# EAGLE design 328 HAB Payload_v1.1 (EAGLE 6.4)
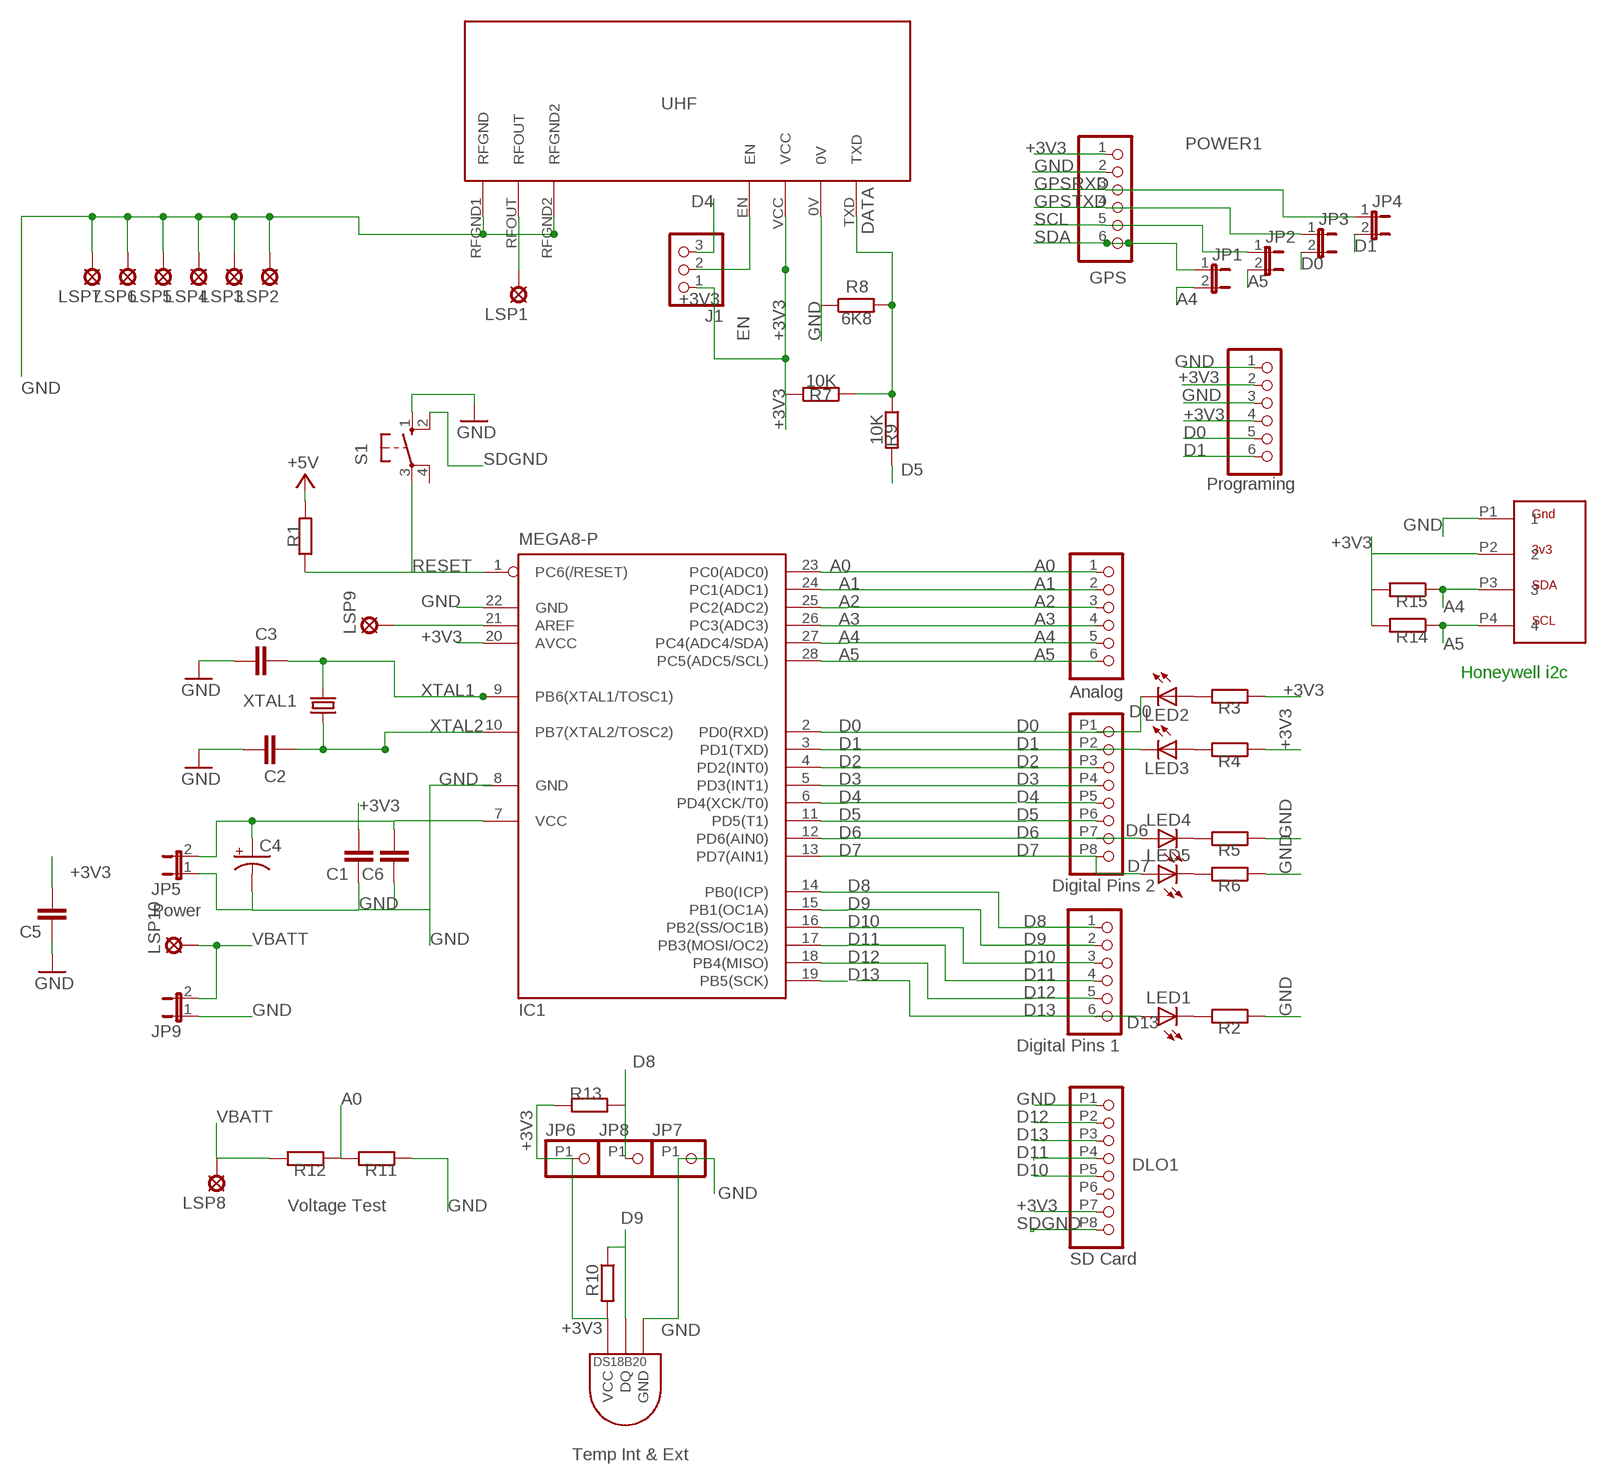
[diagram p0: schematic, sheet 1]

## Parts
ANALOG  PINHD-1X6CLEAN  [1X06-CLEAN]
C1  C-EU025-025X050  [C025-025X050]
C2  C-EU025-025X050  [C025-025X050]
C3  C-EU025-025X050  [C025-025X050]
C4  CAP_POLPTH4  [CPOL-RADIAL-1000UF-25V]
C5  C-EU025-025X050  [C025-025X050]
C6  C-EU025-025X050  [C025-025X050]
DHI  PINHD-1X6CLEAN  [1X06-CLEAN]
DLO  PINHD-1X8  [1X08SMALL]
DLO1  PINHD-1X8  [1X08SMALL]
IC1  MEGA8-P  [DIL28-3]
J1  PINHD-1X3CB  [1X03-CLEANBIG]
JP1  JUMPER-2PTH  [1X02]
JP2  JUMPER-2PTH  [1X02]
JP3  JUMPER-2PTH  [1X02]
JP4  JUMPER-2PTH  [1X02]
JP5  JUMPER-2PTH  [1X02]
JP6  PINHD-1X1UGI  [1X01SML-SQR]
JP7  PINHD-1X1UGI  [1X01SML-SQR]
JP8  PINHD-1X1UGI  [1X01SML-SQR]
JP9  JUMPER-2PTH  [1X02]
LED1  LED3MM  [LED3MM]
LED2  LED3MM  [LED3MM]
LED3  LED3MM  [LED3MM]
LED4  LED3MM  [LED3MM]
LED5  LED3MM  [LED3MM]
LSP1  LSP10  [LSP10]
LSP2  LSP10  [LSP10]
LSP3  LSP13  [LSP13]
LSP4  LSP13  [LSP13]
LSP5  LSP13  [LSP13]
LSP6  LSP13  [LSP13]
LSP7  LSP10  [LSP10]
LSP8  LSP10  [LSP10]
LSP9  LSP10  [LSP10]
LSP10  LSP10  [LSP10]
POWER  PINHD-1X6CLEAN  [1X06-CLEAN]
POWER1  PINHD-1X6CLEAN  [1X06-CLEAN]
R1  R-EU_0207/2V  [0207/2V]
R2  R-EU_0207/2V  [0207/2V]
R3  R-EU_0207/2V  [0207/2V]
R4  R-EU_0207/2V  [0207/2V]
R5  R-EU_0207/2V  [0207/2V]
R6  R-EU_0207/2V  [0207/2V]
R7  10K  R-EU_0207/2V  [0207/2V]
R8  6K8  R-EU_0207/2V  [0207/2V]
R9  10K  R-EU_0207/2V  [0207/2V]
R10  R-EU_0207/2V  [0207/2V]
R11  R-EU_0207/2V  [0207/2V]
R12  R-EU_0207/2V  [0207/2V]
R13  R-EU_0207/2V  [0207/2V]
R14  R-EU_0207/2V  [0207/2V]
R15  R-EU_0207/2V  [0207/2V]
S1  10-XX  [B3F-10XX]
U$1  NTX2-VERTICAL  [NTX2-VERTICAL]
U$2  HSCDANN001BA2A3  [HDC-DIL8]
U$3  DS1820TO92  [DS1820]
XTAL1  CRYTALHC49S  [HC49/S]

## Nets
+3V3 [usbvcc]: C1.2 C4.1(+) C5.2 C6.2 DLO1.P7 IC1.7(VCC) IC1.20(AVCC) J1.1 JP5.2 JP6.P1 POWER1.1 POWER.2 POWER.4 R1.2 R3.1 R4.1 R7.2 R10.2 R13.1 R14.2 R15.2 U$1.VCC U$2.P2 U$3.VDD(VCC) ; supply symbol labelled +5V
A0: ANALOG.1 IC1.23(PC0(ADC0)) R11.2 R12.1
A1: ANALOG.2 IC1.24(PC1(ADC1))
A2: ANALOG.3 IC1.25(PC2(ADC2))
A3: ANALOG.4 IC1.26(PC3(ADC3))
A4: ANALOG.5 IC1.27(PC4(ADC4/SDA)) JP1.2 R15.1 U$2.P3
A5: ANALOG.6 IC1.28(PC5(ADC5/SCL)) JP2.2 R14.1 U$2.P4
AREF: IC1.21(AREF) LSP9.MP
D0: DLO.P1 IC1.2(PD0(RXD)) JP3.2 LED2.K(C) POWER.5
D1: DLO.P2 IC1.3(PD1(TXD)) JP4.2 LED3.K(C) POWER.6
D2: DLO.P3 IC1.4(PD2(INT0))
D3: DLO.P4 IC1.5(PD3(INT1))
D4: DLO.P5 IC1.6(PD4(XCK/T0)) J1.3
D5: DLO.P6 IC1.11(PD5(T1)) R9.2
D6: DLO.P7 IC1.12(PD6(AIN0)) LED4.A
D7: DLO.P8 IC1.13(PD7(AIN1)) LED5.A
D8: DHI.1 IC1.14(PB0(ICP)) JP8.P1 R13.2
D9: DHI.2 IC1.15(PB1(OC1A)) R10.1 U$3.DQ
D10: DHI.3 DLO1.P5 IC1.16(PB2(SS/OC1B))
D11: DHI.4 DLO1.P4 IC1.17(PB3(MOSI/OC2))
D12: DHI.5 DLO1.P2 IC1.18(PB4(MISO))
D13: DHI.6 DLO1.P3 IC1.19(PB5(SCK)) LED1.A
DATA: R7.1 R8.2 R9.1 U$1.TXD
EN: J1.2 U$1.EN
GND [usbvcc]: C1.1 C2.1 C3.1 C4.2(-) C5.1 C6.1 DLO1.P1 IC1.22(GND) JP5.1 JP7.P1 JP9.1 LSP2.MP LSP3.MP LSP4.MP LSP5.MP LSP6.MP LSP7.MP POWER1.2 POWER.1 POWER.3 R2.1 R5.1 R6.1 R8.1 R11.1 S1.1(S) U$1.0V U$1.RFGND1(RFGND) U$1.RFGND2 U$2.P1 U$3.GND
GPSRXD: JP4.1 POWER1.3
GPSTXD: JP3.1 POWER1.4
N$1: LED1.K(C) R2.2
N$2: LED2.A R3.2
N$3: LED3.A R4.2
N$4: LED4.K(C) R5.2
N$5: LED5.K(C) R6.2
N$7: LSP1.MP U$1.RFOUT
RESET: IC1.1(PC6(/RESET)) R1.1 S1.3(P)
SCL: JP2.1 POWER1.5
SDA: JP1.1 POWER1.6
SDGND: DLO1.P8 S1.2(S1)
VBATT: JP9.2 LSP8.MP LSP10.MP R12.2
XTAL1: C3.2 IC1.9(PB6(XTAL1/TOSC1)) XTAL1.2
XTAL2: C2.2 IC1.10(PB7(XTAL2/TOSC2)) XTAL1.1
Unconnected: DLO1.P6 S1.4(P1)

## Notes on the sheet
- UHF
- GPS
- Programing
- Honeywell i2c
- Analog
- Digital Pins 2
- Power
- Digital Pins 1
- Voltage Test
- SD Card
- Temp Int & Ext

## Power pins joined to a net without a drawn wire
GND: IC1.8(GND)

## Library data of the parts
ANALOG DHI POWER POWER1 = adafruit:PINHD-1X6: PIN HEADER
C1-C3 C5 C6 = rcl:C-EU: CAPACITOR, European symbol
C4 = SparkFun:CAP_POL: Capacitor Polarized
DLO DLO1 = UgiLib 2012-11-03:PINHD-1X8: PIN HEADER
IC1 = atmel:MEGA8-P: MICROCONTROLLER 8 Kbytes FLASH, 1 kbytes SRAM, 512 bytes EEPROM, USART, 4-channel 10 bit ADC, 2-channel 8 bit ADC Pin compatible with Atmega48, ATMega88, ATMega168 Source: avr.lbr; OC_FARNELL: unknown; OC_NEWARK: unknown
J1 = adafruit:PINHD-1X3: PIN HEADER
JP1-JP5 JP9 = SparkFun:JUMPER-2: Jumper
JP6-JP8 = UgiLib 2012-11-03:PINHD-1X1: PIN HEADER
LED1-LED5 = led:LED: LED
LSP1 LSP2 LSP7-LSP10 = solpad:LSP10: SOLDER PAD
LSP3-LSP6 = solpad:LSP13: SOLDER PAD
R1-R15 = rcl:R-EU_: RESISTOR, European symbol
S1 = switch-omron:10-XX: OMRON SWITCH; MPN: B3F-1000; OC_FARNELL: 176432; OC_NEWARK: 36M3542
U$1 = Ava:NTX2-VERTICAL: Radiometrix NTX2 Transmitter Module Author Anthony Stirk / http://ava.upuaut.net
U$2 = UgiLib 2012-11-03:HSCDANN001BA2A3: Honeywell HSCDANN001BA2A3 Absolute Pressure Sensor
U$3 = Ava:DS1820: DS18B20 Programmable Resolution 1-Wire Digital Thermometer Description The DS18B20 digital thermometer provides 9-bit to 12-bit Celsius temperature measurements and has an alarm function with nonvolatile user-programmable upper and lower trigger points. The DS18B20 communicates over a 1-Wire® bus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
XTAL1 = crystal:CRYTAL: CRYSTAL

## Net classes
0 default: width 0.254 mm, drill 0.305 mm, clearance 0.152 mm
1 power: width 0.61 mm, drill 0.508 mm, clearance 0.152 mm
2 gnd: width 0.305 mm, drill 0.508 mm, clearance 0.152 mm
3 usbvcc: width 0.508 mm, drill 0.508 mm, clearance 0.152 mm
4 aref: width 0.406 mm

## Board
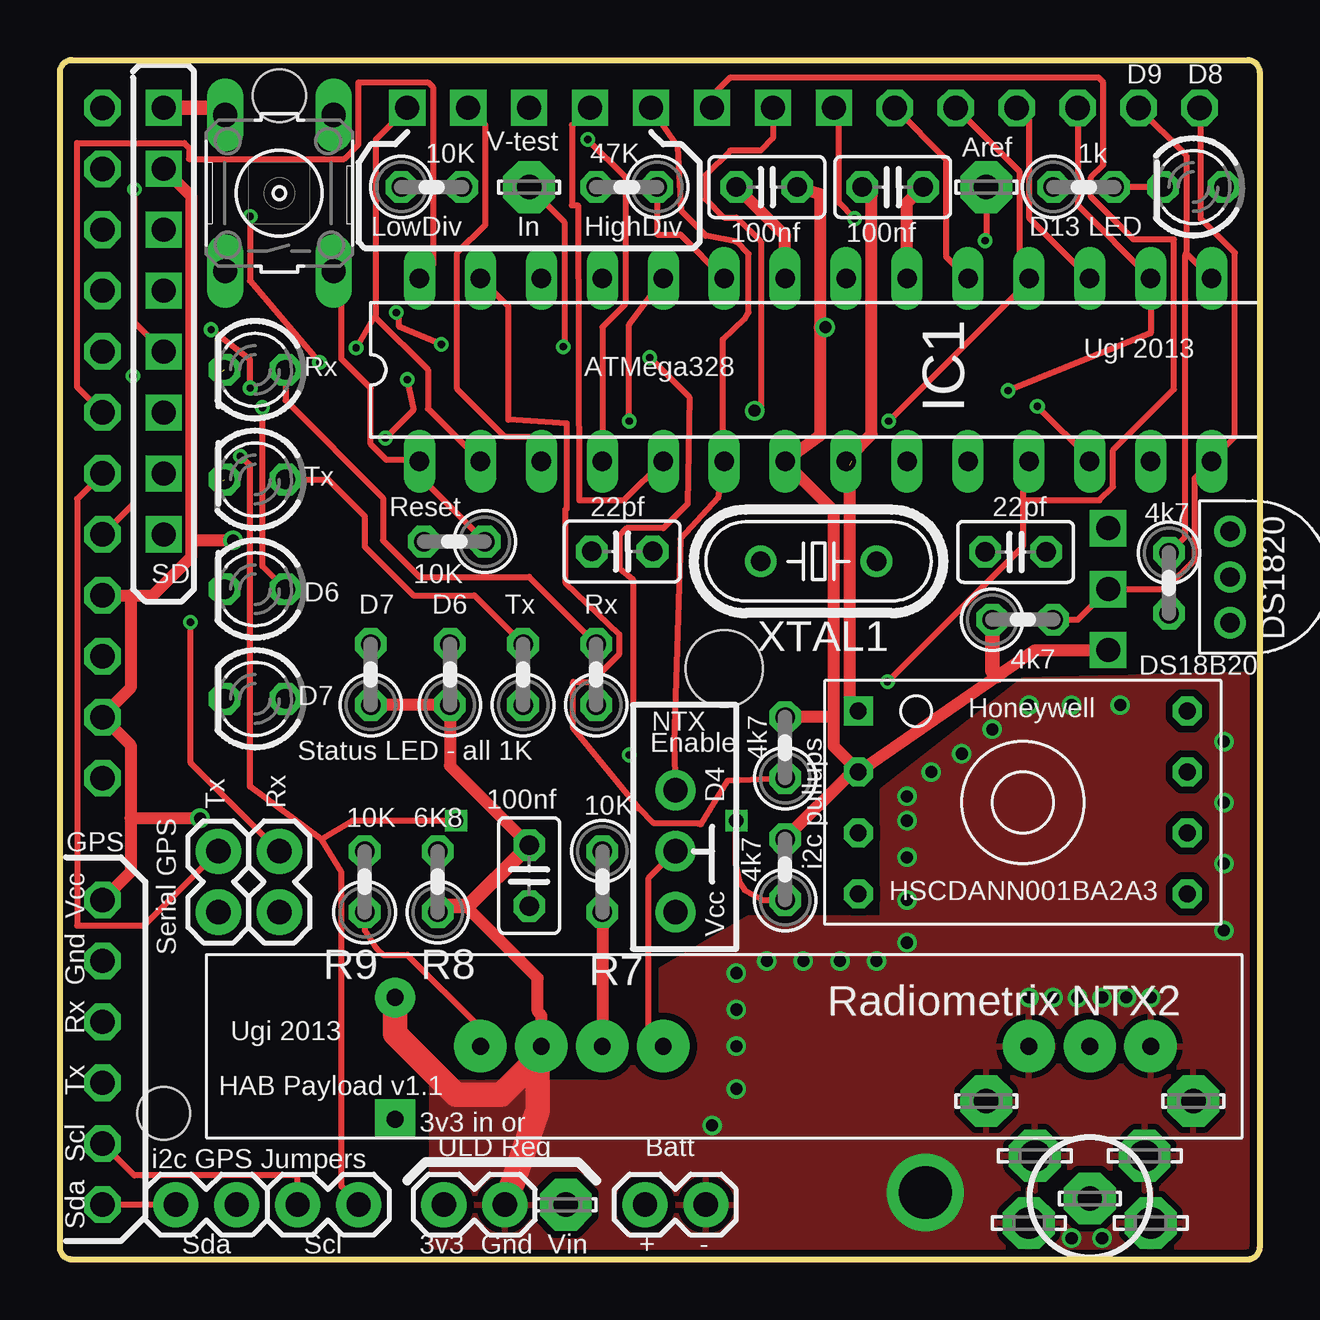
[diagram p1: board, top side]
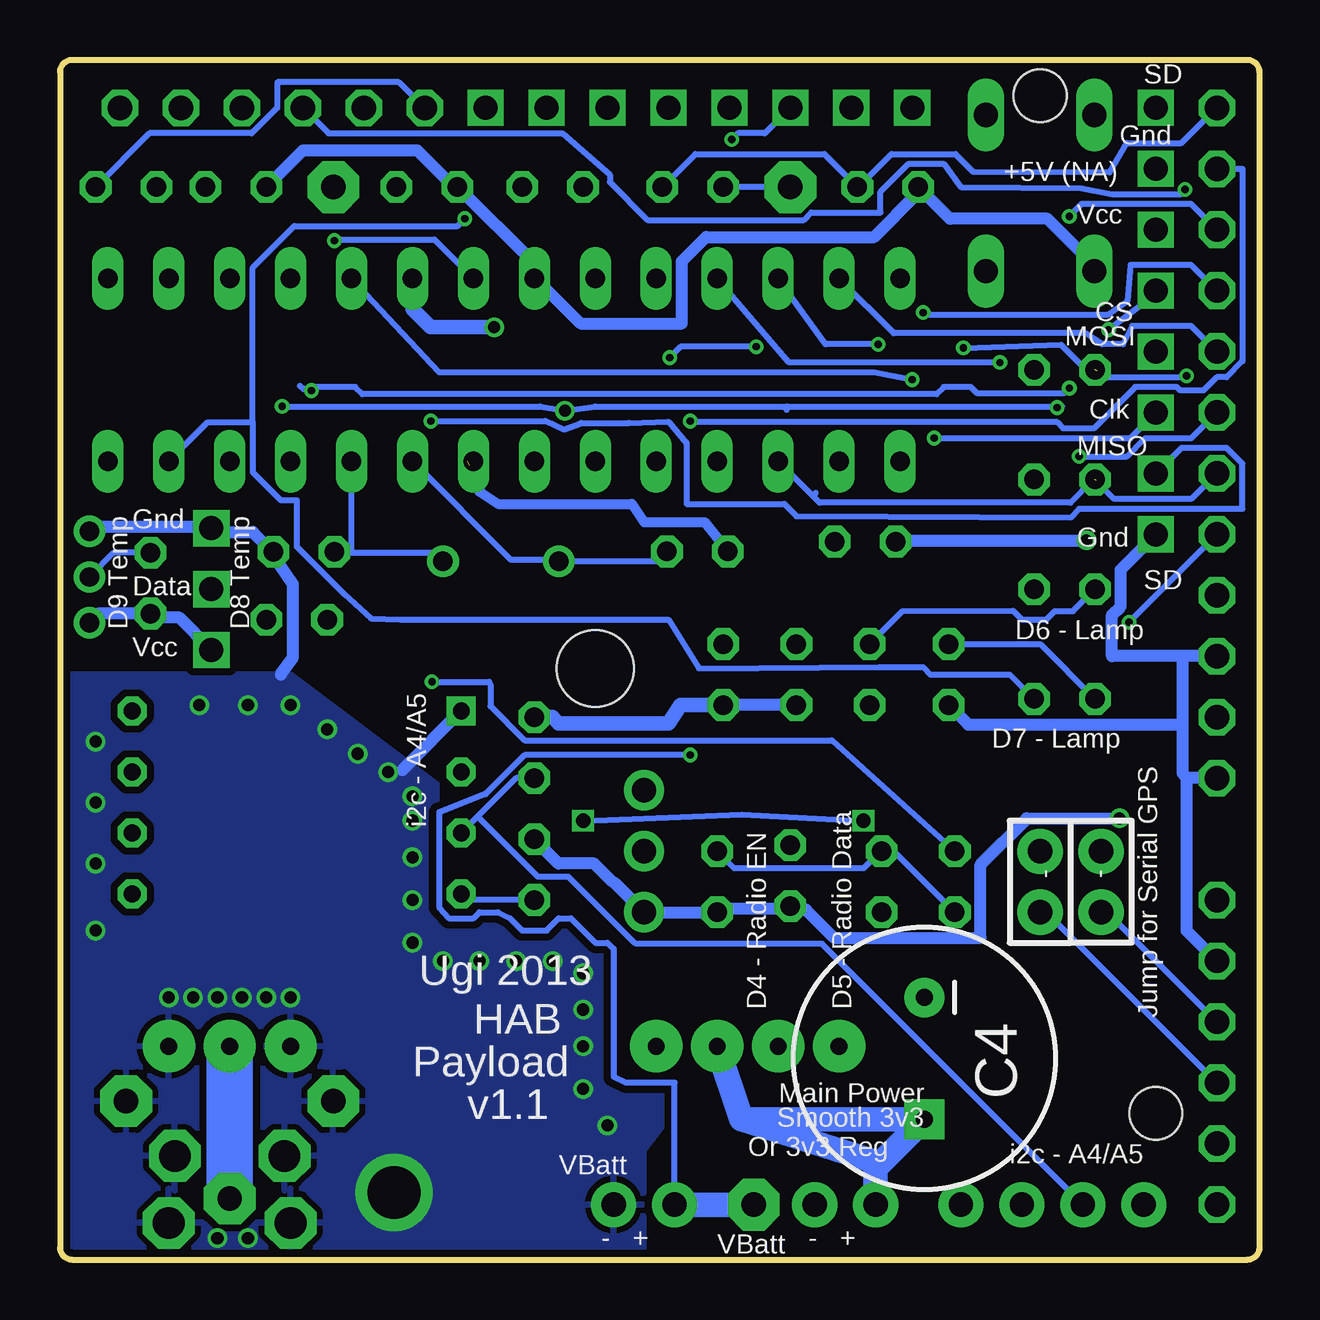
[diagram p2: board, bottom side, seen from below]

Size 50 x 50 mm. Coordinates in mm from the lower left corner, seen from the top.
Outline: 49.5,0 0.5,0 arc-90 0,0.5 0,49.5 arc-90 0.5,50 49.5,50 arc-90 50,49.5 50,0.5 arc-90 49.5,0
Copper layers (1*16): Top 0.035mm / dielectric 1.5mm / Bottom 0.035mm
Design rules "ITEADstudio_DRC": minimum track width 6mil, minimum drill 12mil, track to track 6mil, track to pad 6mil, pad to pad 6mil, via to via 6mil, smd to smd 0mil, copper to edge 10mil, drill to drill 10mil, minimum pad ring 10mil, minimum via ring 6mil, stop-mask expansion 2mil, vias tented up to drill 100mil, thermal gap 10mil
Holes 2.2 mm at 4.32,6.1 9.14,48.51
Holes 3.2 mm at 27.69,24.63

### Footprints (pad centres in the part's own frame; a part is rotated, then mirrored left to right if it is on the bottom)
1X06-CLEAN = drill 1.016 octagon: 1 -6.35,0; 2 -3.81,0; 3 -1.27,0; 4 1.27,0; 5 3.81,0; 6 6.35,0
C025-025X050 = drill 0.813 octagon: 1 -1.27,0; 2 1.27,0
CPOL-RADIAL-1000UF-25V = drill 0.7 pad 1.651 square: 1 2.54,0 | drill 0.7 pad 1.651: 2 -2.54,0
1X08SMALL = drill 1 pad 1.27 square: P1 -8.89,0; P2 -6.35,0; P3 -3.81,0; P4 -1.27,0; P5 1.27,0; P6 3.81,0; P7 6.35,0; P8 8.89,0
DIL28-3 = drill 0.813 long: 1 -16.51,-3.81; 2 -13.97,-3.81; 3 -11.43,-3.81; 4 -8.89,-3.81; 5 -6.35,-3.81; 6 -3.81,-3.81; 7 -1.27,-3.81; 8 1.27,-3.81; 9 3.81,-3.81; 10 6.35,-3.81; 11 8.89,-3.81; 12 11.43,-3.81; 13 13.97,-3.81; 14 16.51,-3.81; 15 16.51,3.81; 16 13.97,3.81; 17 11.43,3.81; 18 8.89,3.81; 19 6.35,3.81; 20 3.81,3.81; 21 1.27,3.81; 22 -1.27,3.81; 23 -3.81,3.81; 24 -6.35,3.81; 25 -8.89,3.81; 26 -11.43,3.81; 27 -13.97,3.81; 28 -16.51,3.81
1X03-CLEANBIG = drill 1.016 pad 1.676: 1 -2.54,0; 2 0,0; 3 2.54,0
1X02 = drill 1.016 pad 1.88: 1 0,0; 2 2.54,0
1X01SML-SQR = drill 1 pad 1.27 square: P1 0,0
LED3MM = drill 0.813 octagon: A -1.27,0; K 1.27,0
LSP10 = drill 1.016 pad 2.159 octagon: MP 0,0
LSP13 = drill 1.321 pad 2.159 octagon: MP 0,0
0207/2V = drill 0.813 octagon: 1 -1.27,0; 2 1.27,0
B3F-10XX = drill 1.016 long: 1 -3.251,2.261; 2 3.251,2.261; 3 -3.251,-2.261; 4 3.251,-2.261
NTX2-VERTICAL = drill 0.7 pad 2.184: 0V 17.78,0; EN 12.7,0; RFGND1 -7.62,0; RFGND2 -2.54,0; RFOUT -5.08,0; TXD 20.32,0; VCC 15.24,0
HDC-DIL8 = drill 0.7 square: P1 -3.81,-6.858 | drill 0.7 octagon: P2 -1.27,-6.858; P3 1.27,-6.858; P4 3.81,-6.858; P5 3.81,6.858; P6 1.27,6.858; P7 -1.27,6.858; P8 -3.81,6.858
DS1820 = drill 0.8: DQ 2.54,-1.27; GND 0.635,-1.27; VDD 4.445,-1.27
HC49/S = drill 0.813: 1 -2.413,0; 2 2.413,0

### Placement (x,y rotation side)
ANALOG  1.78,41.66 270 top
C1  29.46,44.7 0 top
C2  39.83,29.5 180 top
C3  23.43,29.51 0 top
C4  13.97,8.38 270 bottom
C5  34.71,44.7 0 top
C6  19.56,16 270 top
DHI  41.15,48.01 180 top
DLO  23.37,48.01 0 top
DLO1  4.32,39.12 90 top
IC1  31.5,37.08 0 top
J1  25.65,17.02 90 top
JP1  4.83,2.29 0 top
JP2  9.91,2.29 0 top
JP3  9.14,14.48 90 top
JP4  6.6,14.48 90 top
JP5  18.54,2.29 180 top
JP6  43.69,25.4 0 top
JP7  43.69,30.48 0 top
JP8  43.69,27.94 0 top
JP9  26.92,2.29 180 top
LED1  47.24,44.7 180 top
LED2  8.13,37.08 180 top
LED3  8.13,32.51 180 top
LED4  8.13,27.94 180 top
LED5  8.13,23.37 180 top
LSP1  42.93,2.54 0 top
LSP2  38.61,6.6 0 top
LSP3  40.64,4.32 0 top
LSP4  40.39,1.52 0 top
LSP5  45.47,1.52 0 top
LSP6  45.21,4.32 0 top
LSP7  47.24,6.6 0 top
LSP8  19.56,44.7 0 top
LSP9  38.61,44.7 0 top
LSP10  21.08,2.29 0 top
POWER  1.78,26.42 90 top
POWER1  1.78,8.64 270 top
R1  16.44,29.92 180 top
R2  42.67,44.7 0 top
R3  22.35,24.38 90 top
R4  19.3,24.38 90 top
R5  16.26,24.38 90 top
R6  12.95,24.38 90 top
R7  22.61,15.75 270 top
R8  15.75,15.75 90 top
R9  12.7,15.75 90 top
R10  46.23,28.19 270 top
R11  15.49,44.7 0 top
R12  23.62,44.7 180 top
R13  40.13,26.67 0 top
R14  30.23,16.26 90 top
R15  30.23,21.34 90 top
S1  9.14,44.45 90 top
U$1  37.85,8.89 180 top
U$2  40.13,19.05 270 top
U$3  50.04,30.99 270 top
XTAL1  31.62,29.1 180 top

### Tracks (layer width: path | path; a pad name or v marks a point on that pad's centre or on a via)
+3V3  (via drill 0.51)
  Top 0.508: POWER1.1 2.95,16.15 2.95,18.39 | 2.95,18.39 2.95,21.44 POWER.2 1.93,22.81 2.95,23.82 2.95,27.69 | DLO1.P7 5.49,44.3 5.49,29.97 | 5.49,29.97 5.49,29.31 3.86,27.69 2.95,27.69 | POWER.4 2.95,27.69 | 31.67,38.86 31.67,44.4 C1.2 | 31.67,38.86 31.67,34.34 IC1.7 30.38,33.07 32.26,31.19 32.26,22.61 | 15.19,29.92 R1.2 | R7.2 U$1.VCC | JP6.P1 40.64,25.4 39.08,24.32 U$2.P2 | 32.26,22.61 32.26,21.39 33.12,20.52 U$2.P2 | v7.21,29.97 5.49,29.97 | v5.84,18.39 2.95,18.39 | v31.9,38.86 31.67,38.86 | IC1.20 35.31,44.04 35.97,44.7 C5.2 | R14.2 32.97,20.27 32.97,20.32 U$2.P2 | 32.26,22.61 R15.2
  Top 0.61: R13.1 38.86,24.54 39.08,24.32
  Bottom 0.508: U$3.VDD 48.77,26.57 48.41,26.92 R10.2 46.02,26.77 45.06,26.77 JP6.P1 | v7.21,29.97 15.14,29.97 R1.2 | v5.84,18.39 9.7,18.39 11.63,16.46 11.63,13.41 17.73,13.41 18.9,14.58 19.36,14.58 C6.2 19.66,14.63 22.4,14.63 R7.2 J1.1 26.82,15.65 27.03,15.8 27.74,16.51 29.21,16.51 R14.2 | v31.9,38.86 31.93,38.86 | R4.1 R3.1
  Bottom 0.61: IC1.20 35.31,39.62 34.54,38.86 31.93,38.86 | R3.1 24.13,23.11 24.64,22.35 29.21,22.35 29.46,22.61 R15.2
  Bottom 1.016: 21.59,5.84 C4.1 16,3.81 JP5.2 | 21.59,5.84 16,4.06 | U$1.VCC 21.59,5.84
A0
  Top 0.254: IC1.23 25.86,42.72 24.89,42.72 R12.1
  Bottom 0.254: R12.1 23.52,46.08 18.14,46.08 R11.2 16.66,44.76 15.34,46.08 12.68,46.08 11.94,45.34 6.25,45.31 5.54,46.53 3.25,46.53 ANALOG.1
A1  (via drill 0.3)
  Top 0.254: IC1.24 23.72,38.96 v23.72,34.95
  Bottom 0.254: v23.72,34.95 23.93,34.9 8.43,34.9 8.18,34.65 6.91,34.65 5.18,36.37 3.45,36.37 3.3,36.22 2.34,36.22 1.78,36.78 1.37,36.78 0.71,37.44 0.71,45.47 ANALOG.2
A2  (via drill 0.3)
  Top 0.254: v10.82,37.39 7.92,40.79 v7.92,43.48
  Bottom 0.254: IC1.25 19.61,37.39 v10.82,37.39 | v7.92,43.48 7.42,43.99 2.85,43.99 ANALOG.3
A3  (via drill 0.3)
  Top 0.254: v15.9,38.15 14.12,38.91 14.12,39.37 v14.02,39.47
  Bottom 0.254: IC1.26 18.09,38.15 v15.9,38.15 | v14.02,39.47 13.92,39.37 6.33,39.37 5.51,39.93 5.38,41.45 2.85,41.45 ANALOG.4
A4
  Top 0.254: IC1.27 18.69,39.73 18.69,35 21.13,34.85 21.13,31.29 21.08,31.29 21.08,28.19 23.32,26.06 23.32,25.25 22.15,24.08 21.39,24.08 21.39,22.15 24.13,18.8 24.74,18.19 26.62,18.19 26.72,18.14 27.84,19.96 R15.1
  Bottom 0.254: IC1.27 15.24,38.61 7.26,38.61 6.55,38.15 5.69,38.15 5.31,38.91 2.85,38.91 ANALOG.5 | JP1.2 18.24,13.16 25.96,13.16 26.06,13.21 28.8,15.95 30.07,15.95 32.59,18.47 | 32.59,18.47 30.99,20.07 R15.1 | 32.59,18.47 U$2.P3
A5  (via drill 0.3, 0.6)
  Top 0.254: IC1.28 15.54,41.45 15.54,48.87 15.34,49.07 12.45,49.07 12.45,46.48 11.84,45.87 5.38,45.87 5.38,46.33 5.18,46.53 0.71,46.53 0.71,36.37 ANALOG.6 | v7.52,33.48 7.92,33.12 7.92,19.71 10.9,17.5 | 10.9,17.5 11.73,16.15 11.73,3.05 12.39,2.39 JP2.2 | R14.1 29.31,14.99 28.55,15.39 28.35,15.7 28.17,16.48 28.17,17.5 v28.19,18.29 | v16.51,18.29 12.19,18.29 10.9,17.5
  Bottom 0.254: ANALOG.6 2.85,34.24 4.78,34.24 5.54,33.48 v7.52,33.48 | U$2.P4 33.02,14.99 R14.1 | v28.19,18.29 21.59,18.54 v16.51,18.29
AREF  (via drill 0.3)
  Top 0.254: v38.56,42.47 38.61,42.52 LSP9.MP
  Bottom 0.254: IC1.21 34.39,42.52 38.51,42.52 v38.56,42.47
D0  (via drill 0.3)  (1 unrouted)
  Top 0.254: IC1.2 15.34,35.46 15.34,37.08 13.16,39.27 | 13.16,39.27 13.16,46.69 DLO.P1 | v12.34,38 13.06,39.22 13.16,39.27 | POWER.5 3.05,31.5 v3.05,36.83 | JP3.2 5.44,20.73 v5.44,26.57
  Bottom 0.254: v12.34,38 8.28,38.12 7.24,37.08 LED2.K | v3.05,36.83 3.1,36.78 6.5,36.78 6.76,37.03 | POWER.5 v5.44,26.57
D1  (1 unrouted)
  Top 0.254: DLO.P2 17.73,47.3 17.73,43.13 16.56,41.96 16.56,36.27 18.49,34.34 18.59,34.29 20.07,34.29 IC1.3 | JP4.2 3.5,13.92 0.71,13.92 0.71,31.7 POWER.6
  Bottom 0.254: POWER.6 2.85,31.7 6.04,31.7 6.81,32.46 6.96,32.46 7.87,31.55 18.34,31.55 18.62,31.83 | 18.62,31.83 IC1.3 | 18.49,31.95 18.62,31.83
D2  (via drill 0.3)
  Top 0.254: IC1.4 22.61,38.86 23.57,39.83 23.57,45.11 v22,46.69
  Bottom 0.254: v22,46.69 21.74,46.94 20.62,46.94 DLO.P3
D3
  Top 0.254: IC1.5 23.52,31.65 21.64,31.65 21.59,43.94 21.34,43.94 21.34,47.3 21.39,47.3 DLO.P4
D4
  Top 0.254: DLO.P5 25.76,46.38 25.91,43.69 26.92,42.67 28.19,42.42 28.7,41.91 28.7,39.47 28.55,39.22 27.64,38.35 27.64,33.38 IC1.6 27.64,33.17 27.43,31.75 25.86,30.02 25.6,21.54 J1.3
D5  (via drill 0.3)
  Top 0.254: v34.49,24.08 40.13,29.72 40.13,31.65 | 40.13,31.65 40.13,33.02 IC1.11 | 40.13,31.65 43.33,31.65 43.89,32.21 43.89,33.73 46.43,36.27 46.43,42.52 44.76,42.52 42.98,44.3 42.98,45.11 43.48,45.62 43.48,49.07 43.28,49.28 27.94,49.28 27.18,48.51 DLO.P6
  Bottom 0.254: R9.2 17.83,21.64 30.63,21.64 32.05,23.06 32.05,23.98 32.11,24.08 v34.49,24.08
D6  (via drill 0.3, 0.5)
  Top 0.254: v8.43,35.51 8.43,28.91 LED4.A | v40.74,35.56 42.93,33.38 IC1.12 | DLO.P7 29.72,46.74 29.21,46.23 27.94,46.23 26.92,45.21 26.92,44.2 27.69,43.43 28.19,43.43 29.21,42.42 29.21,35.56 v28.96,35.38
  Bottom 0.254: v8.43,35.51 8.23,35.56 19.71,35.56 | v40.74,35.56 29.97,35.56 v28.96,35.38 27.69,35.56 19.71,35.56 | 19.71,35.41 19.71,35.56
D7  (via drill 0.3)
  Top 0.254: DLO.P8 32.46,47.8 32.46,44.04 v33.12,43.38
  Bottom 0.254: 41.96,34.9 41.96,32.82 40.79,31.65 40.13,31.65 40.13,29.72 38.15,27.74 37.03,26.72 35.81,26.67 24.64,26.67 23.37,24.64 15.85,24.69 14.02,24.69 13.72,24.38 10.41,24.38 LED5.A | 41.96,34.9 43.84,34.9 IC1.13 | v33.12,43.38 33.43,43.08 40.23,43.08 41.96,41.35 41.96,34.9
D8
  Top 0.254: DHI.1 47.55,47.95 47.55,43.38 48.97,41.96 48.97,34.29 48.06,33.38 IC1.14 47.3,32.56 47.3,29.16 46.08,27.94 JP8.P1 42.42,26.67 R13.2
D9
  Top 0.254: 46.97,41.94 46.94,41.96 46.94,46.02 DHI.2 | 46.97,41.94 IC1.15 | R10.1 46.89,30.12 46.89,41.86 46.97,41.94
  Bottom 0.254: U$3.DQ 47.75,29.46 R10.1
D10  (via drill 0.3)
  Top 0.254: DHI.3 42.42,43.94 IC1.16 45.26,40.95 45.47,40.95 45.47,38.61 v39.52,36.22 | v6.3,38.76 7.92,37.52 v7.92,36.32
  Bottom 0.254: DLO1.P5 4.88,39.83 6.25,38.81 v6.3,38.76 | v7.92,36.32 8.13,36.12 11.79,36.12 12.04,36.37 13.16,36.37 13.46,36.07 37.39,36.07 37.69,36.37 39.37,36.37 v39.52,36.22 39.62,36.27 39.83,36.27 39.88,36.32 39.96,36.37 39.99,36.41
D11  (via drill 0.3)
  Top 0.254: IC1.17 40.39,43.43 40.39,47.5 DHI.4 | DLO1.P4 3.1,39.06 v3.1,44.6
  Bottom 0.254: v3.1,44.6 3.3,44.4 6.15,44.4 7.42,44.65 12.45,44.7 13.16,45.67 14.63,45.67 15.8,44.5 15.8,43.64 18.69,43.64 19,43.33 25.5,43.33 27.08,44.91 27.08,45.21 29.06,46.94 38.81,46.94 DHI.4
D12  (via drill 0.3)
  Top 0.254: DHI.5 39.98,45.36 39.98,41.3 IC1.18 40.34,40.79 40.34,40.74 v34.54,34.95
  Bottom 0.254: DLO1.P2 3.25,33.83 1.37,33.83 0.71,33.17 0.71,31.29 7.52,31.29 7.87,30.94 19.3,30.99 19.81,31.5 23.88,31.5 23.88,34.04 24.64,34.92 26.29,34.87 28.27,34.87 29.01,34.59 29.77,34.95 v34.54,34.95
D13  (via drill 0.3)
  Top 0.254: IC1.19 36.93,41.81 36.93,45.87 DHI.6 | v13.56,34.24 14.73,35.41 v14.48,36.68
  Bottom 0.254: LED1.A 46.28,46.94 42.01,46.94 40.95,48.01 40.95,49.07 35.87,49.07 DHI.6 | DLO1.P3 5.38,34.24 v13.56,34.24 | v14.48,36.68 16.05,36.98 34.19,36.98 IC1.19
DATA
  Top 0.254: U$1.TXD 17.53,9.65 14.48,12.7 13.46,12.7 13.21,12.95 12.7,13.72 R9.1
  Bottom 0.254: R9.1 15.24,17.02 R8.2 15.85,16.97 16.51,16.31 21.89,16.31 R7.1
EN
  Top 0.254: J1.2 24.54,15.9 24.54,9.5 U$1.EN
GND  (via drill 0.51, 2.2)  (1 unrouted)
  Top 0.406: 32.92,23.22 33.02,23.22
  Top 0.508: R6.1 R5.1 16.26,20.57 C6.1 | 19.3,17.53 C6.1 | 22.15,29.46 C3.1 | C1.1 30.23,42.67 IC1.22 | 19.91,8.69 U$1.0V 20.07,10.16 19.91,10.36 19.91,11.73 17.17,14.48 17.02,14.73 | U$2.P1 32.92,23.22 32.92,33.12 IC1.8 32.92,33.48 33.83,34.39 33.83,44.35 33.48,44.7 C5.1 | 19.71,17.07 C6.1 | R8.1 16,14.73
  Top 0.61: 19.71,17.07 19.36,17.07 17.02,14.73 16,14.73
  Top 1.016: JP5.1 19.91,6.2 19.91,8.38 | 19.91,8.69 19.91,8.38 | C4.2 13.97,9.4 16.51,6.86 18.39,6.86 19.91,8.38
  Bottom 0.406: 33.02,33.27 32.51,33.27 32.51,32 31.75,31.5 26.16,31.5 25.65,30.73 23.13,30.73 C3.1
  Bottom 0.508: DLO1.P1 5.79,28.75 5.79,27.23 6.15,26.87 6.15,25.15 3.2,25.15 | POWER.3 3.2,25.15 | POWER1.2 3.05,13.72 3.05,20.07 | POWER.1 3.05,20.07 | 3.2,22.3 3.2,20.27 3.05,20.07 | 3.2,22.3 3.2,25.15 | 3.2,22.3 12.14,22.3 R6.1 | S1.1 6.91,41.45 8.84,43.38 12.9,43.38 R11.1 14.28,44.4 16.05,42.62 23.06,42.62 24.08,41.6 24.08,39.01 28.3,39.01 30.02,40.74 IC1.22 30.23,41.5 33.43,44.7 C5.1 33.68,44.81 35.1,46.23 39.88,46.23 R2.1 | U$3.GND 48.77,30.38 48.62,30.53 43.74,30.53 JP7.P1 43.48,30.33 41.96,30.33 41.15,29.52 C2.1 41.05,29.26 40.28,28.14 40.28,25.09 40.79,24.38 | U$2.P1 35.66,20.47 35.73,20.39
  other vias: 40.39,10.92 41.4,10.92 42.42,10.92 43.43,10.92 44.45,10.92 45.47,10.92 42.16,0.89 43.43,0.89 36.07,2.79 27.18,5.59 28.19,7.11 28.19,8.89 28.19,10.41 28.19,11.94 29.46,12.45 30.99,12.45 32.51,12.45 34.04,12.45 35.31,13.21 35.31,14.99 35.31,16.76 35.31,18.29 35.31,19.3 36.32,20.32 37.59,21.08 38.86,22.1 40.39,23.11 42.16,23.11 44.2,23.11 48.51,21.59 48.51,19.05 48.51,16.51 48.51,13.72
  pour Top (isolate 0.305): 15.49,0.51 49.53,0.51 49.53,24.38 40.13,24.13 34.29,19.56 34.29,14.22 28.7,14.22 23.11,10.92 23.11,7.37 15.49,7.37
  pour Bottom (isolate 0.305): 25.65,0.51 25.65,4.57 23.88,6.86 23.88,11.43 29.21,14.48 34.29,14.48 34.29,19.81 40.39,24.38 49.53,24.38 49.53,0.51
GPSRXD
  Bottom 0.254: POWER1.3 6.35,14.48 JP4.1
GPSTXD
  Bottom 0.254: POWER1.4 8.89,14.48 JP3.1
N$1
  Top 0.254: LED1.K R2.2
N$2
  Top 0.254: LED2.A 9.4,35.81 13.46,31.75 13.46,29.97 14.99,28.45 19.56,28.45 R3.2
N$3
  Top 0.254: LED3.A 11.18,32.51 12.7,30.99 12.7,29.72 14.73,27.69 17.27,27.69 R4.2
N$4
  Bottom 0.254: R5.2 14.88,27.03 10.29,27.05 9.91,26.67 8.89,26.67 8.53,27.03 7.77,27.03 LED4.K
N$5
  Bottom 0.254: R6.2 9.14,25.65 LED5.K
N$7
  Bottom 1.93: U$1.RFOUT LSP1.MP
RESET
  Top 0.254: R1.1 17.68,29.97 14.99,32.66 IC1.1 14.88,33.33 13.61,33.33 12.95,33.98 12.95,36.32 11.73,37.54 11.73,41.15 11.43,41.45 S1.3
SCL
  Top 0.254: POWER1.5 3.1,3.5 9.91,3.5 JP2.1
SDA
  Top 0.254: JP1.1 POWER1.6
SDGND
  Top 0.61: DLO1.P8 6.88,48.01 S1.2
VBATT  (via drill 0.3)
  Top 0.254: v23.72,21.03 23.88,21.18 23.88,28.35 23.32,28.8 23.32,30.18 23.62,30.48 25.15,30.48 26.16,31.5 26.24,35.94 v24.59,37.59 | v20.98,38.05 21.03,38.1 21.03,43.23 LSP8.MP
  Bottom 0.254: LSP8.MP R12.2 | v23.72,21.03 30.63,21.03 32.26,19.41 34.19,18.64 34.19,14.68 33.78,14.22 32.77,14.22 32.51,14.48 31.75,14.48 31.24,14.22 30.73,13.72 29.72,13.72 29.21,14.22 28.7,14.22 27.69,13.21 27.18,13.21 26.92,12.95 26.92,7.62 26.42,7.37 24.38,7.37 JP9.2 | v24.59,37.59 24.13,38.05 v20.98,38.05
  Bottom 1.016: LSP10.MP JP9.2
XTAL1
  Bottom 0.254: C3.2 24.74,29.46 25.09,29.11 29.16,29.11 XTAL1.2 29.31,29.16 31.19,29.16 IC1.9
XTAL2
  Bottom 0.254: 37.85,29.46 38.56,29.46 C2.2 | 37.85,29.46 34.39,29.46 XTAL1.1 | 37.85,29.46 IC1.10

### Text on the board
tNames: D9 | D8 | 10K | V-test | 47K | Aref | 1k | LowDiv | In | HighDiv | D13 LED | 100nf | 100nf | Ugi 2013 | Rx | ATMega328 | Tx | Reset | 22pf | 22pf | 4k7 | SD | 10K | D6 | D7 | D6 | Tx | Rx | 4k7 | DS18B20 | D7 | NTX | Honeywell | Enable | Status LED - all 1K | 4k7 | Tx | Rx | 100nf | 10K | D4 | 10K | 6K8 | GPS | 4k7 | i2c pullups | HSCDANN001BA2A3 | Vcc | Serial GPS | Vcc | Gnd | Rx | Ugi 2013 | Tx | HAB Payload v1.1 | 3v3 in or | Scl | i2c GPS Jumpers | ULD Reg | Batt | Sda | Sda | Scl | 3v3 | Gnd | Vin | + | -
bNames: SD | Gnd | +5V (NA) | Vcc | CS | MOSI | Clk | MISO | D8 Temp | D9 Temp | Gnd | Gnd | SD | Data | D6 - Lamp | Vcc | i2c - A4/A5 | Jump for Serial GPS | D7 - Lamp | - | - | Ugi 2013 | D5 - Radio Data | D4 - Radio EN | HAB | Payload | Main Power | Smooth 3v3 | v1.1 | i2c - A4/A5 | Or 3v3 Reg | VBatt | - + | - + | VBatt
bStop: To / V-Test
tMap: D0 | D1 | D2 | D3 | D4 | D5 | D6 | D7 | 13 | 12 | 11 | 10 | A0 | A1 | A2 | A3 | A4 | A5 | Tx | Rx | Vcc | Gnd | Vcc | Gnd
